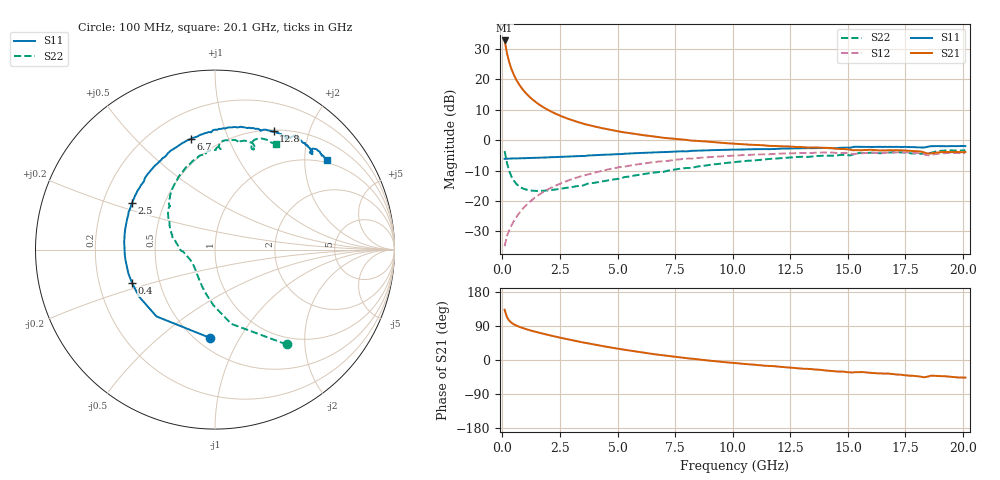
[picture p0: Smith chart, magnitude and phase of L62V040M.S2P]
!  Infineon Technologies AG
! BFR380L3 , PF131585-7, No.6, Th 09.10.01, soldered on pcb-board, measured with PP GSG850
!  Vce=2.0 V,  Ic=40.0 mA
! Common Emitter S-Parameters:  15. November 2001
#  GHz  S  MA  R  50
! f  S11  S21  S12  S22
! GHz  Mag  Ang  Mag  Ang  Mag  Ang  Mag  Ang
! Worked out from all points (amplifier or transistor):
!   201 points, 100 MHz to 20.1 GHz, reference 50 ohm
!   highest |S21| = 32.7 dB at 100 MHz (marker M1)
!   |S21| within 3 dB of that: start of sweep to 173 MHz
!   unconditionally stable (mu >= 1): 996.3 MHz to 4.29 GHz
!   at 3.4 GHz: K = 1.02, MAG = 8.0 dB, |S12| = -11.9 dB
!   at 10.1 GHz: K = 0.96, MSG = 1.9 dB, |S12| = -5.1 dB
!   at 20.1 GHz: K = 0.99, MSG = 0.1 dB, |S12| = -4.2 dB
!   S11 on the Smith chart (normalised r, x): 100 MHz: 0.58, -0.76; 400 MHz: 0.35, -0.17; 2.5 GHz: 0.33, +0.24; 6.7 GHz: 0.36, +0.74; 12.8 GHz: 0.51, +1.48; 20.1 GHz: 0.94, +2.56
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0.1  0.4925 -93.3  43.26 132.7  0.01815 59.6  0.6623 -52.9
0.2  0.4949 -131.3  26.96 113.0  0.02643 57.7  0.4238 -77.6
0.3  0.4975 -148.2  19.03 103.9  0.03337 59.5  0.3109 -91.5
0.4  0.4982 -158.1  14.59 98.3  0.03988 61.7  0.2511 -101.6
0.5  0.5007 -164.6  11.81 94.2  0.04662 64.3  0.2157 -109.7
0.6  0.5002 -169.7  9.905 91.2  0.05369 65.8  0.193 -116.3
0.7  0.5023 -173.6  8.537 88.5  0.06085 66.8  0.1781 -122.1
0.8  0.5034 -176.9  7.501 86.1  0.06828 67.7  0.1677 -127.0
1  0.5053 177.4  6.038 82.1  0.08297 68.5  0.1553 -135.1
1.3  0.5105 170.8  4.682 76.7  0.1051 68.4  0.1479 -144.2
1.6  0.5145 165.1  3.836 71.9  0.1273 67.4  0.1467 -151.1
2  0.5204 158.2  3.103 66.0  0.1564 65.4  0.15 -158.3
2.5  0.531 150.5  2.524 59.0  0.1919 62.5  0.158 -165.7
3.5  0.5486 136.6  1.868 46.3  0.2611 55.6  0.1797 -176.9
5.1  0.5881 118.0  1.38 28.8  0.3602 43.8  0.2333 165.6
6.7  0.6324 102.5  1.13 14.5  0.44 32.6  0.2966 148.6
6.8  0.6338 101.3  1.119 13.6  0.4454 31.7  0.2987 147.6
10.1  0.6985 77.4  0.8722 -8.1  0.5576 10.1  0.436 120.2
12.8  0.7367 63.7  0.7695 -21.8  0.6127 -6.2  0.53 99.5
13.5  0.7379 60.3  0.7566 -24.7  0.6177 -10.1  0.541 95.3
16.8  0.7754 48.1  0.6848 -36.1  0.6233 -25.5  0.6251 75.7
20.1  0.7973 38.5  0.6388 -46.5  0.6175 -39.0  0.6796 60.3
